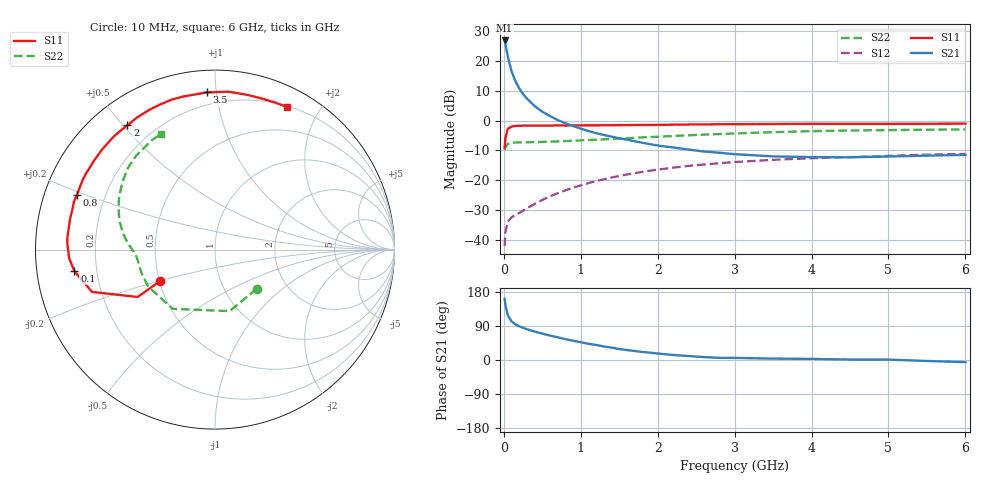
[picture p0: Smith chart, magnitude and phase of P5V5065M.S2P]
! SIEMENS Small Signal Semiconductors
! BFP183
! Si NPN RF Bipolar Junction Transistor in SOT143
! VCE = 0.5 V  IC = 65 mA
! Common Emitter S-Parameters:  March  1996
# GHz  S  MA  R  50
!  f  S11  S21  S12  S22
! GHz  MAG  ANG  MAG  ANG  MAG  ANG  MAG  ANG
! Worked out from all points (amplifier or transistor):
!   36 points, 10 MHz to 6 GHz, reference 50 ohm
!   highest |S21| = 26.9 dB at 10 MHz (marker M1)
!   |S21| within 3 dB of that: start of sweep to 33.89 MHz
!   unconditionally stable (mu >= 1): start of sweep to 41.81 MHz; 80.45 MHz to end of sweep
!   at 250 MHz: K = 1.73, MAG = 14.6 dB, |S12| = -30.3 dB
!   at 1.4 GHz: K = 2.19, MAG = 0.7 dB, |S12| = -19.1 dB
!   at 6 GHz: K = 1.37, MAG = -3.8 dB, |S12| = -11.2 dB
!   S11 on the Smith chart (normalised r, x): 10 MHz: 0.50, -0.20; 100 MHz: 0.12, -0.08; 800 MHz: 0.10, +0.19; 2 GHz: 0.10, +0.51; 3.5 GHz: 0.12, +0.94; 6 GHz: 0.21, +1.60
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0.01  0.3526 -150.2  22.17 161.6  0.0078 54.0  0.3194 -43.2
0.02  0.5053 -148.5  19.64 145.8  0.0133 49.4  0.3523 -76.7
0.05  0.7246 -161.0  12.1 118.8  0.02 37.3  0.4058 -125.6
0.1  0.7926 -171.3  6.733 102.0  0.0238 31.4  0.425 -151.1
0.15  0.814 -176.7  4.608 94.1  0.0262 34.4  0.4286 -160.7
0.2  0.8188 180.0  3.476 89.0  0.0282 38.7  0.4311 -165.6
0.25  0.8241 177.3  2.8 84.7  0.0307 42.6  0.432 -168.5
0.3  0.8251 175.2  2.34 81.2  0.0338 45.5  0.433 -170.6
0.4  0.8236 171.3  1.758 75.1  0.0398 50.2  0.4364 -173.3
0.5  0.8254 167.9  1.41 69.7  0.0466 53.4  0.4397 -175.1
0.6  0.8253 164.5  1.192 64.4  0.0535 55.1  0.4434 -176.5
0.7  0.8302 161.3  1.023 59.9  0.0604 56.4  0.448 -177.7
0.8  0.8275 158.3  0.904 55.1  0.0674 56.4  0.4525 -178.7
1.1  0.8346 149.6  0.669 42.7  0.0893 55.8  0.4716 178.2
1.5  0.8406 138.8  0.505 28.8  0.1176 52.0  0.499 173.6
2  0.8471 125.2  0.382 17.1  0.1502 45.3  0.5356 166.9
2.2  0.8545 120.6  0.354 13.3  0.1624 42.3  0.5533 163.6
2.8  0.8695 106.4  0.289 5.7  0.1927 33.3  0.5956 154.3
3.5  0.8771 93.0  0.251 3.7  0.2195 23.8  0.6397 143.7
4.5  0.8805 78.0  0.242 1.2  0.2443 11.8  0.6827 130.2
5.5  0.885 67.8  0.258 -2.6  0.2683 2.1  0.7038 119.9
6  0.8902 63.3  0.266 -5.7  0.2752 -2.9  0.7113 115.2
